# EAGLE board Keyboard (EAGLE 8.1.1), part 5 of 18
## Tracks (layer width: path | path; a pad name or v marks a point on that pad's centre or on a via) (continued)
S$4259 (continued)
  Bottom 0: 29.64,10.47 29.58,10.45
S$4260
  Bottom 0: 29.58,10.45 29.52,10.41
S$4261
  Bottom 0: 29.52,10.41 29.47,10.37
S$4262
  Bottom 0: 29.47,10.37 22.33,3.23
S$4263
  Bottom 0: 22.33,3.23 18.7,3.23
S$4264
  Bottom 0: 21.59,6.04 22.1,6.04
S$4265
  Bottom 0: 22.1,6.04 22.61,6.12
S$4266
  Bottom 0: 22.61,6.12 23.11,6.29
S$4267
  Bottom 0: 23.11,6.29 23.56,6.54
S$4268
  Bottom 0: 23.56,6.54 23.97,6.86
S$4269
  Bottom 0: 23.97,6.86 24.32,7.24
S$4270
  Bottom 0: 24.32,7.24 24.61,7.67
S$4271
  Bottom 0: 24.61,7.67 24.81,8.15
S$4272
  Bottom 0: 24.81,8.15 24.94,8.64
S$4273
  Bottom 0: 24.94,8.64 24.98,9.16
S$4274
  Bottom 0: 24.98,9.16 24.94,9.68
S$4275
  Bottom 0: 24.94,9.68 24.81,10.18
S$4276
  Bottom 0: 24.81,10.18 24.61,10.65
S$4277
  Bottom 0: 24.61,10.65 24.32,11.09
S$4278
  Bottom 0: 24.32,11.09 23.97,11.47
S$4279
  Bottom 0: 23.97,11.47 23.56,11.79
S$4280
  Bottom 0: 23.56,11.79 23.11,12.03
S$4281
  Bottom 0: 23.11,12.03 22.61,12.2
S$4282
  Bottom 0: 22.61,12.2 22.1,12.29
S$4283
  Bottom 0: 22.1,12.29 21.59,12.29
S$4284
  Bottom 0: 21.59,12.29 21.08,12.2
S$4285
  Bottom 0: 21.08,12.2 20.59,12.03
S$4286
  Bottom 0: 20.59,12.03 20.13,11.79
S$4287
  Bottom 0: 20.13,11.79 19.72,11.47
S$4288
  Bottom 0: 19.72,11.47 19.37,11.09
S$4289
  Bottom 0: 19.37,11.09 19.09,10.65
S$4290
  Bottom 0: 19.09,10.65 18.88,10.18
S$4291
  Bottom 0: 18.88,10.18 18.75,9.68
S$4292
  Bottom 0: 18.75,9.68 18.71,9.16
S$4293
  Bottom 0: 18.71,9.16 18.75,8.64
S$4294
  Bottom 0: 18.75,8.64 18.88,8.15
S$4295
  Bottom 0: 18.88,8.15 19.09,7.67
S$4296
  Bottom 0: 19.09,7.67 19.37,7.24
S$4297
  Bottom 0: 19.37,7.24 19.72,6.86
S$4298
  Bottom 0: 19.72,6.86 20.13,6.54
S$4299
  Bottom 0: 20.13,6.54 20.59,6.29
S$4300
  Bottom 0: 20.59,6.29 21.08,6.12
S$4301
  Bottom 0: 21.08,6.12 21.59,6.04
S$4302
  Bottom 0: 31.59,11.49 33.37,11.49
S$4303
  Bottom 0: 33.37,11.49 33.44,11.5
S$4304
  Bottom 0: 33.44,11.5 33.51,11.54
S$4305
  Bottom 0: 33.51,11.54 33.57,11.6
S$4306
  Bottom 0: 33.57,11.6 33.61,11.67
S$4307
  Bottom 0: 33.61,11.67 33.62,11.75
S$4308
  Bottom 0: 33.62,11.75 33.62,13.53
S$4309
  Bottom 0: 33.62,13.53 33.61,13.6
S$4310
  Bottom 0: 33.61,13.6 33.57,13.67
S$4311
  Bottom 0: 33.57,13.67 33.51,13.73
S$4312
  Bottom 0: 33.51,13.73 33.44,13.77
S$4313
  Bottom 0: 33.44,13.77 33.37,13.78
S$4314
  Bottom 0: 33.37,13.78 31.59,13.78
S$4315
  Bottom 0: 31.59,13.78 31.51,13.77
S$4316
  Bottom 0: 31.51,13.77 31.44,13.73
S$4317
  Bottom 0: 31.44,13.73 31.39,13.67
S$4318
  Bottom 0: 31.39,13.67 31.35,13.6
S$4319
  Bottom 0: 31.35,13.6 31.34,13.53
S$4320
  Bottom 0: 31.34,13.53 31.34,11.75
S$4321
  Bottom 0: 31.34,11.75 31.35,11.67
S$4322
  Bottom 0: 31.35,11.67 31.39,11.6
S$4323
  Bottom 0: 31.39,11.6 31.44,11.54
S$4324
  Bottom 0: 31.44,11.54 31.51,11.5
S$4325
  Bottom 0: 31.51,11.5 31.59,11.49
S$4326
  Bottom 0: 206.63,3.26 205.49,4.4
S$4327
  Bottom 0: 205.49,4.4 205.6,4.67
S$4328
  Bottom 0: 205.6,4.67 205.65,5.02
S$4329
  Bottom 0: 205.65,5.02 205.6,5.36
S$4330
  Bottom 0: 205.6,5.36 205.47,5.69
S$4331
  Bottom 0: 205.47,5.69 205.26,5.97
S$4332
  Bottom 0: 205.26,5.97 205,6.2
S$4333
  Bottom 0: 205,6.2 204.69,6.34
S$4334
  Bottom 0: 204.69,6.34 204.69,11.95
S$4335
  Bottom 0: 204.69,11.95 204.68,12.02
S$4336
  Bottom 0: 204.68,12.02 204.67,12.09
S$4337
  Bottom 0: 204.67,12.09 204.65,12.15
S$4338
  Bottom 0: 204.65,12.15 204.6,12.21
S$4339
  Bottom 0: 204.6,12.21 204.56,12.27
S$4340
  Bottom 0: 204.56,12.27 197.05,19.77
S$4341
  Bottom 0: 197.05,19.77 197,19.81
S$4342
  Bottom 0: 197,19.81 196.94,19.85
S$4343
  Bottom 0: 196.94,19.85 196.88,19.88
S$4344
  Bottom 0: 196.88,19.88 196.81,19.89
S$4345
  Bottom 0: 196.81,19.89 196.74,19.9
S$4346
  Bottom 0: 196.74,19.9 192.38,19.9
S$4347
  Bottom 0: 192.38,19.9 188.82,23.45
S$4348
  Bottom 0: 188.82,23.45 188.93,23.72
S$4349
  Bottom 0: 188.93,23.72 188.97,24.07
S$4350
  Bottom 0: 188.97,24.07 188.93,24.41
S$4351
  Bottom 0: 188.93,24.41 188.8,24.74
S$4352
  Bottom 0: 188.8,24.74 188.59,25.02
S$4353
  Bottom 0: 188.59,25.02 188.32,25.25
S$4354
  Bottom 0: 188.32,25.25 188.01,25.4
S$4355
  Bottom 0: 188.01,25.4 187.66,25.46
S$4356
  Bottom 0: 187.66,25.46 187.31,25.44
S$4357
  Bottom 0: 187.31,25.44
S$4358
  Bottom 0: 187.31,25.44 192.08,30.21
S$4359
  Bottom 0: 192.08,30.21 192.39,30.21
S$4360
  Bottom 0: 192.39,30.21 192.56,29.96
S$4361
  Bottom 0: 192.56,29.96 192.8,29.77
S$4362
  Bottom 0: 192.8,29.77 193.08,29.66
S$4363
  Bottom 0: 193.08,29.66 193.38,29.64
S$4364
  Bottom 0: 193.38,29.64 193.68,29.7
S$4365
  Bottom 0: 193.68,29.7 193.94,29.86
S$4366
  Bottom 0: 193.94,29.86 194.14,30.08
S$4367
  Bottom 0: 194.14,30.08 194.27,30.35
S$4368
  Bottom 0: 194.27,30.35 194.32,30.65
S$4369
  Bottom 0: 194.32,30.65 194.27,30.95
S$4370
  Bottom 0: 194.27,30.95 194.14,31.22
S$4371
  Bottom 0: 194.14,31.22 193.94,31.44
S$4372
  Bottom 0: 193.94,31.44 193.68,31.59
S$4373
  Bottom 0: 193.68,31.59 193.38,31.66
S$4374
  Bottom 0: 193.38,31.66 193.21,31.65
S$4375
  Bottom 0: 193.21,31.65 197.37,35.82
S$4376
  Bottom 0: 197.37,35.82 198.23,35.82
S$4377
  Bottom 0: 198.23,35.82 198.1,35.69
S$4378
  Bottom 0: 198.1,35.69 197.93,35.41
S$4379
  Bottom 0: 197.93,35.41 197.84,35.1
S$4380
  Bottom 0: 197.84,35.1 197.84,34.77
S$4381
  Bottom 0: 197.84,34.77 197.93,34.46
S$4382
  Bottom 0: 197.93,34.46 198.1,34.19
S$4383
  Bottom 0: 198.1,34.19 198.33,33.96
S$4384
  Bottom 0: 198.33,33.96 198.62,33.81
S$4385
  Bottom 0: 198.62,33.81 198.95,33.75
S$4386
  Bottom 0: 198.95,33.75 199.27,33.77
S$4387
  Bottom 0: 199.27,33.77 199.49,33.85
S$4388
  Bottom 0: 199.49,33.85 200.55,32.8
S$4389
  Bottom 0: 200.55,32.8 200.51,32.78
S$4390
  Bottom 0: 200.51,32.78 200.45,32.72
S$4391
  Bottom 0: 200.45,32.72 200.41,32.65
S$4392
  Bottom 0: 200.41,32.65 200.4,32.58
S$4393
  Bottom 0: 200.4,32.58 200.4,30.8
S$4394
  Bottom 0: 200.4,30.8 200.41,30.72
S$4395
  Bottom 0: 200.41,30.72 200.45,30.65
S$4396
  Bottom 0: 200.45,30.65 200.51,30.59
S$4397
  Bottom 0: 200.51,30.59 200.58,30.55
S$4398
  Bottom 0: 200.58,30.55 200.66,30.54
S$4399
  Bottom 0: 200.66,30.54 202.44,30.54
S$4400
  Bottom 0: 202.44,30.54 202.51,30.55
S$4401
  Bottom 0: 202.51,30.55 202.58,30.59
S$4402
  Bottom 0: 202.58,30.59 202.64,30.65
S$4403
  Bottom 0: 202.64,30.65 202.68,30.72
S$4404
  Bottom 0: 202.68,30.72 202.69,30.8
S$4405
  Bottom 0: 202.69,30.8 202.69,32.58
S$4406
  Bottom 0: 202.69,32.58 202.68,32.64
S$4407
  Bottom 0: 202.68,32.64 203.09,32.23
S$4408
  Bottom 0: 203.09,32.23 202.99,32.01
S$4409
  Bottom 0: 202.99,32.01 202.94,31.69
S$4410
  Bottom 0: 202.94,31.69 202.99,31.37
S$4411
  Bottom 0: 202.99,31.37 203.13,31.07
S$4412
  Bottom 0: 203.13,31.07 203.34,30.82
S$4413
  Bottom 0: 203.34,30.82 203.61,30.64
S$4414
  Bottom 0: 203.61,30.64 203.92,30.55
S$4415
  Bottom 0: 203.92,30.55 204.25,30.55
S$4416
  Bottom 0: 204.25,30.55 204.56,30.64
S$4417
  Bottom 0: 204.56,30.64 204.83,30.82
S$4418
  Bottom 0: 204.83,30.82 205.05,31.07
S$4419
  Bottom 0: 205.05,31.07 205.18,31.37
S$4420
  Bottom 0: 205.18,31.37 205.23,31.69
S$4421
  Bottom 0: 205.23,31.69 205.18,32.01
S$4422
  Bottom 0: 205.18,32.01 205.05,32.31
S$4423
  Bottom 0: 205.05,32.31 204.83,32.55
S$4424
  Bottom 0: 204.83,32.55 204.56,32.73
S$4425
  Bottom 0: 204.56,32.73 204.25,32.82
S$4426
  Bottom 0: 204.25,32.82 204.1,32.82
S$4427
  Bottom 0: 204.1,32.82 200.13,36.79
S$4428
  Bottom 0: 200.13,36.79 200.07,36.85
S$4429
  Bottom 0: 200.07,36.85 199.99,36.89
S$4430
  Bottom 0: 199.99,36.89 199.91,36.93
S$4431
  Bottom 0: 199.91,36.93 199.82,36.95
S$4432
  Bottom 0: 199.82,36.95 199.73,36.95
S$4433
  Bottom 0: 199.73,36.95 199.51,36.95
S$4434
  Bottom 0: 199.51,36.95 199.51,46.35
S$4435
  Bottom 0: 199.51,46.35 199.51,46.44
S$4436
  Bottom 0: 199.51,46.44 199.49,46.53
S$4437
  Bottom 0: 199.49,46.53 199.45,46.61
S$4438
  Bottom 0: 199.45,46.61 199.41,46.69
S$4439
  Bottom 0: 199.41,46.69 199.35,46.75
S$4440
  Bottom 0: 199.35,46.75 195.66,50.43
S$4441
  Bottom 0: 195.66,50.43 195.7,50.74
S$4442
  Bottom 0: 195.7,50.74 195.66,51.06
S$4443
  Bottom 0: 195.66,51.06 195.52,51.36
S$4444
  Bottom 0: 195.52,51.36 195.31,51.6
S$4445
  Bottom 0: 195.31,51.6 195.03,51.78
S$4446
  Bottom 0: 195.03,51.78 195,51.79
S$4447
  Bottom 0: 195,51.79 195.25,51.79
S$4448
  Bottom 0: 195.25,51.79 206.08,40.96
S$4449
  Bottom 0: 206.08,40.96 206.08,35.97
S$4450
  Bottom 0: 206.08,35.97 205.95,35.91
S$4451
  Bottom 0: 205.95,35.91 205.72,35.69
S$4452
  Bottom 0: 205.72,35.69 205.55,35.41
S$4453
  Bottom 0: 205.55,35.41 205.46,35.1
S$4454
  Bottom 0: 205.46,35.1 205.46,34.77
S$4455
  Bottom 0: 205.46,34.77 205.55,34.46
S$4456
  Bottom 0: 205.55,34.46 205.72,34.19
S$4457
  Bottom 0: 205.72,34.19 205.95,33.96
S$4458
  Bottom 0: 205.95,33.96 206.08,33.9
S$4459
  Bottom 0: 206.08,33.9 206.08,27.1
S$4460
  Bottom 0: 206.08,27.1 205.02,26.04
S$4461
  Bottom 0: 205.02,26.04 205.06,26.16
S$4462
  Bottom 0: 205.06,26.16 205.1,26.61
S$4463
  Bottom 0: 205.1,26.61 205.06,27.05
S$4464
  Bottom 0: 205.06,27.05 204.93,27.48
S$4465
  Bottom 0: 204.93,27.48 204.72,27.88
S$4466
  Bottom 0: 204.72,27.88 204.43,28.22
S$4467
  Bottom 0: 204.43,28.22 204.09,28.51
S$4468
  Bottom 0: 204.09,28.51 203.69,28.72
S$4469
  Bottom 0: 203.69,28.72 203.26,28.85
S$4470
  Bottom 0: 203.26,28.85 202.82,28.89
S$4471
  Bottom 0: 202.82,28.89 202.37,28.85
S$4472
  Bottom 0: 202.37,28.85 201.94,28.72
S$4473
  Bottom 0: 201.94,28.72 201.55,28.51
S$4474
  Bottom 0: 201.55,28.51 201.2,28.22
S$4475
  Bottom 0: 201.2,28.22 200.92,27.88
S$4476
  Bottom 0: 200.92,27.88 200.7,27.48
S$4477
  Bottom 0: 200.7,27.48 200.58,27.05
S$4478
  Bottom 0: 200.58,27.05 200.53,26.61
S$4479
  Bottom 0: 200.53,26.61 200.58,26.16
S$4480
  Bottom 0: 200.58,26.16 200.7,25.73
S$4481
  Bottom 0: 200.7,25.73 200.92,25.34
S$4482
  Bottom 0: 200.92,25.34 201.2,24.99
S$4483
  Bottom 0: 201.2,24.99 201.55,24.71
S$4484
  Bottom 0: 201.55,24.71 201.94,24.49
S$4485
  Bottom 0: 201.94,24.49 202.37,24.37
S$4486
  Bottom 0: 202.37,24.37 202.82,24.32
S$4487
  Bottom 0: 202.82,24.32 203.26,24.37
S$4488
  Bottom 0: 203.26,24.37 203.69,24.49
S$4489
  Bottom 0: 203.69,24.49 203.7,24.5
S$4490
  Bottom 0: 203.7,24.5 203.7,16.92
S$4491
  Bottom 0: 203.7,16.92 203.58,16.86
S$4492
  Bottom 0: 203.58,16.86 203.34,16.64
S$4493
  Bottom 0: 203.34,16.64 203.17,16.36
S$4494
  Bottom 0: 203.17,16.36 203.09,16.05
S$4495
  Bottom 0: 203.09,16.05 203.09,15.72
S$4496
  Bottom 0: 203.09,15.72 203.17,15.41
S$4497
  Bottom 0: 203.17,15.41 203.34,15.14
S$4498
  Bottom 0: 203.34,15.14 203.58,14.91
S$4499
  Bottom 0: 203.58,14.91 203.87,14.77
S$4500
  Bottom 0: 203.87,14.77 204.19,14.7
S$4501
  Bottom 0: 204.19,14.7 204.51,14.72
S$4502
  Bottom 0: 204.51,14.72 204.81,14.83
S$4503
  Bottom 0: 204.81,14.83 205.08,15.01
S$4504
  Bottom 0: 205.08,15.01 205.29,15.27
S$4505
  Bottom 0: 205.29,15.27 205.42,15.57
S$4506
  Bottom 0: 205.42,15.57 205.46,15.89
S$4507
  Bottom 0: 205.46,15.89 205.42,16.21
S$4508
  Bottom 0: 205.42,16.21 205.29,16.51
S$4509
  Bottom 0: 205.29,16.51 205.08,16.76
S$4510
  Bottom 0: 205.08,16.76 204.84,16.93
S$4511
  Bottom 0: 204.84,16.93 204.84,24.25
S$4512
  Bottom 0: 204.84,24.25 207.05,26.46
S$4513
  Bottom 0: 207.05,26.46 207.11,26.53
S$4514
  Bottom 0: 207.11,26.53 207.16,26.61
S$4515
  Bottom 0: 207.16,26.61 207.19,26.69
S$4516
  Bottom 0: 207.19,26.69 207.21,26.78
S$4517
  Bottom 0: 207.21,26.78 207.22,26.87
S$4518
  Bottom 0: 207.22,26.87 207.22,33.89
S$4519
  Bottom 0: 207.22,33.89 207.46,34.06
S$4520
  Bottom 0: 207.46,34.06 207.57,34.2
S$4521
  Bottom 0: 207.57,34.2 207.57,25.64
S$4522
  Bottom 0: 207.57,25.64 207.24,25.31
S$4523
  Bottom 0: 207.24,25.31 207.06,25.4
S$4524
  Bottom 0: 207.06,25.4 206.71,25.46
S$4525
  Bottom 0: 206.71,25.46 206.36,25.44
S$4526
  Bottom 0: 206.36,25.44 206.03,25.33
S$4527
  Bottom 0: 206.03,25.33 205.74,25.14
S$4528
  Bottom 0: 205.74,25.14 205.5,24.89
S$4529
  Bottom 0: 205.5,24.89 205.32,24.58
S$4530
  Bottom 0: 205.32,24.58 205.24,24.24
S$4531
  Bottom 0: 205.24,24.24 205.24,23.89
S$4532
  Bottom 0: 205.24,23.89 205.32,23.55
S$4533
  Bottom 0: 205.32,23.55 205.5,23.24
S$4534
  Bottom 0: 205.5,23.24 205.74,22.99
S$4535
  Bottom 0: 205.74,22.99 206.03,22.8
S$4536
  Bottom 0: 206.03,22.8 206.36,22.7
S$4537
  Bottom 0: 206.36,22.7 206.71,22.68
S$4538
  Bottom 0: 206.71,22.68 207.06,22.74
S$4539
  Bottom 0: 207.06,22.74 207.24,22.82
S$4540
  Bottom 0: 207.24,22.82 219.15,10.92
S$4541
  Bottom 0: 219.15,10.92 219.21,10.88
S$4542
  Bottom 0: 219.21,10.88 219.27,10.84
S$4543
  Bottom 0: 219.27,10.84 219.33,10.81
S$4544
  Bottom 0: 219.33,10.81 219.39,10.8
S$4545
  Bottom 0: 219.39,10.8 219.46,10.79
S$4546
  Bottom 0: 219.46,10.79 224.05,10.79
S$4547
  Bottom 0: 224.05,10.79 225.25,9.6
S$4548
  Bottom 0: 225.25,9.6 225.12,9.67
S$4549
  Bottom 0: 225.12,9.67 224.7,9.8
S$4550
  Bottom 0: 224.7,9.8 224.25,9.84
S$4551
  Bottom 0: 224.25,9.84 223.8,9.8
S$4552
  Bottom 0: 223.8,9.8 223.38,9.67
S$4553
  Bottom 0: 223.38,9.67 222.98,9.46
S$4554
  Bottom 0: 222.98,9.46 222.63,9.17
S$4555
  Bottom 0: 222.63,9.17 222.35,8.83
S$4556
  Bottom 0: 222.35,8.83 222.14,8.43
S$4557
  Bottom 0: 222.14,8.43 222.01,8
S$4558
  Bottom 0: 222.01,8 221.96,7.56
S$4559
  Bottom 0: 221.96,7.56 222.01,7.11
S$4560
  Bottom 0: 222.01,7.11 222.14,6.68
S$4561
  Bottom 0: 222.14,6.68 222.35,6.29
S$4562
  Bottom 0: 222.35,6.29 222.63,5.94
S$4563
  Bottom 0: 222.63,5.94 222.98,5.66
S$4564
  Bottom 0: 222.98,5.66 223.38,5.44
S$4565
  Bottom 0: 223.38,5.44 223.8,5.32
S$4566
  Bottom 0: 223.8,5.32 224.25,5.27
S$4567
  Bottom 0: 224.25,5.27 224.7,5.32
S$4568
  Bottom 0: 224.7,5.32 225.12,5.44
S$4569
  Bottom 0: 225.12,5.44 225.52,5.66
S$4570
  Bottom 0: 225.52,5.66 225.86,5.94
S$4571
  Bottom 0: 225.86,5.94 226.15,6.29
S$4572
  Bottom 0: 226.15,6.29 226.36,6.68
S$4573
  Bottom 0: 226.36,6.68 226.49,7.11
S$4574
  Bottom 0: 226.49,7.11 226.53,7.56
S$4575
  Bottom 0: 226.53,7.56 226.49,8
S$4576
  Bottom 0: 226.49,8 226.36,8.43
S$4577
  Bottom 0: 226.36,8.43 226.3,8.55
S$4578
  Bottom 0: 226.3,8.55 227.62,7.23
S$4579
  Bottom 0: 227.62,7.23 227.62,6.33
S$4580
  Bottom 0: 227.62,6.33 227.47,6.28
S$4581
  Bottom 0: 227.47,6.28 227.17,6.09
S$4582
  Bottom 0: 227.17,6.09 226.93,5.84
S$4583
  Bottom 0: 226.93,5.84 226.76,5.53
S$4584
  Bottom 0: 226.76,5.53 226.67,5.19
S$4585
  Bottom 0: 226.67,5.19 226.67,4.84
S$4586
  Bottom 0: 226.67,4.84 226.76,4.5
S$4587
  Bottom 0: 226.76,4.5 226.93,4.19
S$4588
  Bottom 0: 226.93,4.19 227.17,3.94
S$4589
  Bottom 0: 227.17,3.94 227.27,3.88
S$4590
  Bottom 0: 227.27,3.88 225.16,3.88
S$4591
  Bottom 0: 225.16,3.88 224.66,4.39
S$4592
  Bottom 0: 224.66,4.39 224.6,4.43
S$4593
  Bottom 0: 224.6,4.43 224.54,4.47
S$4594
  Bottom 0: 224.54,4.47 224.48,4.49
S$4595
  Bottom 0: 224.48,4.49 224.41,4.51
S$4596
  Bottom 0: 224.41,4.51 224.34,4.51
S$4597
  Bottom 0: 224.34,4.51 217.05,4.51
S$4598
  Bottom 0: 217.05,4.51 216.97,4.51
S$4599
  Bottom 0: 216.97,4.51 216.91,4.49
S$4600
  Bottom 0: 216.91,4.49 216.84,4.46
S$4601
  Bottom 0: 216.84,4.46 216.79,4.43
S$4602
  Bottom 0: 216.79,4.43 216.73,4.38
S$4603
  Bottom 0: 216.73,4.38 215.62,3.26
S$4604
  Bottom 0: 215.62,3.26 215.46,3.26
S$4605
  Bottom 0: 215.46,3.26 215.58,3.4
S$4606
  Bottom 0: 215.58,3.4 215.72,3.67
S$4607
  Bottom 0: 215.72,3.67 215.76,3.98
S$4608
  Bottom 0: 215.76,3.98 215.72,4.28
S$4609
  Bottom 0: 215.72,4.28 215.58,4.55
S$4610
  Bottom 0: 215.58,4.55 215.38,4.77
S$4611
  Bottom 0: 215.38,4.77 215.12,4.92
S$4612
  Bottom 0: 215.12,4.92 214.82,4.99
S$4613
  Bottom 0: 214.82,4.99 214.52,4.97
S$4614
  Bottom 0: 214.52,4.97 214.24,4.85
S$4615
  Bottom 0: 214.24,4.85 214,4.67
S$4616
  Bottom 0: 214,4.67 213.83,4.42
S$4617
  Bottom 0: 213.83,4.42 213.74,4.13
S$4618
  Bottom 0: 213.74,4.13 213.74,3.82
S$4619
  Bottom 0: 213.74,3.82 213.83,3.53
S$4620
  Bottom 0: 213.83,3.53 214,3.28
S$4621
  Bottom 0: 214,3.28 214.02,3.26
S$4622
  Bottom 0: 214.02,3.26 206.63,3.26
S$4623
  Bottom 0: 214.82,10.58 215.12,10.65
S$4624
  Bottom 0: 215.12,10.65 215.38,10.8
S$4625
  Bottom 0: 215.38,10.8 215.58,11.02
S$4626
  Bottom 0: 215.58,11.02 215.72,11.29
S$4627
  Bottom 0: 215.72,11.29 215.76,11.6
S$4628
  Bottom 0: 215.76,11.6 215.72,11.89
S$4629
  Bottom 0: 215.72,11.89 215.58,12.17
S$4630
  Bottom 0: 215.58,12.17 215.38,12.39
S$4631
  Bottom 0: 215.38,12.39 215.12,12.54
S$4632
  Bottom 0: 215.12,12.54 214.82,12.61
S$4633
  Bottom 0: 214.82,12.61 214.52,12.59
S$4634
  Bottom 0: 214.52,12.59 214.24,12.47
S$4635
  Bottom 0: 214.24,12.47 214,12.29
S$4636
  Bottom 0: 214,12.29 213.83,12.04
S$4637
  Bottom 0: 213.83,12.04 213.74,11.75
S$4638
  Bottom 0: 213.74,11.75 213.74,11.44
S$4639
  Bottom 0: 213.74,11.44 213.83,11.15
S$4640
  Bottom 0: 213.83,11.15 214,10.9
S$4641
  Bottom 0: 214,10.9 214.24,10.72
S$4642
  Bottom 0: 214.24,10.72 214.52,10.6
S$4643
  Bottom 0: 214.52,10.6 214.82,10.58
S$4644
  Bottom 0: 200.36,20.14 200.71,20.2
S$4645
  Bottom 0: 200.71,20.2 201.02,20.35
S$4646
  Bottom 0: 201.02,20.35 201.29,20.57
S$4647
  Bottom 0: 201.29,20.57 201.5,20.86
S$4648
  Bottom 0: 201.5,20.86 201.63,21.18
S$4649
  Bottom 0: 201.63,21.18 201.67,21.53
S$4650
  Bottom 0: 201.67,21.53 201.63,21.87
S$4651
  Bottom 0: 201.63,21.87 201.5,22.2
S$4652
  Bottom 0: 201.5,22.2 201.29,22.48
S$4653
  Bottom 0: 201.29,22.48 201.02,22.7
S$4654
  Bottom 0: 201.02,22.7 200.71,22.86
S$4655
  Bottom 0: 200.71,22.86 200.36,22.92
S$4656
  Bottom 0: 200.36,22.92 200.01,22.9
S$4657
  Bottom 0: 200.01,22.9 199.68,22.79
S$4658
  Bottom 0: 199.68,22.79 199.66,22.78
S$4659
  Bottom 0: 199.66,22.78 199.09,23.34
S$4660
  Bottom 0: 199.09,23.34 199.03,23.39
S$4661
  Bottom 0: 199.03,23.39 198.97,23.43
S$4662
  Bottom 0: 198.97,23.43 198.91,23.45
S$4663
  Bottom 0: 198.91,23.45 198.84,23.47
S$4664
  Bottom 0: 198.84,23.47 198.77,23.47
S$4665
  Bottom 0: 198.77,23.47 194.21,23.47
S$4666
  Bottom 0: 194.21,23.47 194.14,23.6
S$4667
  Bottom 0: 194.14,23.6 193.94,23.82
S$4668
  Bottom 0: 193.94,23.82 193.68,23.98
S$4669
  Bottom 0: 193.68,23.98 193.38,24.04
S$4670
  Bottom 0: 193.38,24.04 193.08,24.02
S$4671
  Bottom 0: 193.08,24.02 192.8,23.91
S$4672
  Bottom 0: 192.8,23.91 192.56,23.72
S$4673
  Bottom 0: 192.56,23.72 192.39,23.47
S$4674
  Bottom 0: 192.39,23.47 192.3,23.18
S$4675
  Bottom 0: 192.3,23.18 192.3,22.88
S$4676
  Bottom 0: 192.3,22.88 192.39,22.59
S$4677
  Bottom 0: 192.39,22.59 192.56,22.34
S$4678
  Bottom 0: 192.56,22.34 192.8,22.15
S$4679
  Bottom 0: 192.8,22.15 193.08,22.04
S$4680
  Bottom 0: 193.08,22.04 193.38,22.02
S$4681
  Bottom 0: 193.38,22.02 193.68,22.09
S$4682
  Bottom 0: 193.68,22.09 193.94,22.24
S$4683
  Bottom 0: 193.94,22.24 194.14,22.46
S$4684
  Bottom 0: 194.14,22.46 194.21,22.59
S$4685
  Bottom 0: 194.21,22.59 198.59,22.59
S$4686
  Bottom 0: 198.59,22.59 199.03,22.14
S$4687
  Bottom 0: 199.03,22.14 198.97,22.04
S$4688
  Bottom 0: 198.97,22.04 198.89,21.7
S$4689
  Bottom 0: 198.89,21.7 198.89,21.35
S$4690
  Bottom 0: 198.89,21.35 198.97,21.01
S$4691
  Bottom 0: 198.97,21.01 199.15,20.7
S$4692
  Bottom 0: 199.15,20.7 199.39,20.45
S$4693
  Bottom 0: 199.39,20.45 199.68,20.26
S$4694
  Bottom 0: 199.68,20.26 200.01,20.16
S$4695
  Bottom 0: 200.01,20.16 200.36,20.14
S$4696
  Bottom 0: 202.91,41.07 203.21,41.13
S$4697
  Bottom 0: 203.21,41.13 203.47,41.28
S$4698
  Bottom 0: 203.47,41.28 203.67,41.51
S$4699
  Bottom 0: 203.67,41.51 203.81,41.78
S$4700
  Bottom 0: 203.81,41.78 203.85,42.08
S$4701
  Bottom 0: 203.85,42.08 203.81,42.38
S$4702
  Bottom 0: 203.81,42.38 203.67,42.65
S$4703
  Bottom 0: 203.67,42.65 203.47,42.87
S$4704
  Bottom 0: 203.47,42.87 203.21,43.02
S$4705
  Bottom 0: 203.21,43.02 202.91,43.09
S$4706
  Bottom 0: 202.91,43.09 202.61,43.07
S$4707
  Bottom 0: 202.61,43.07 202.33,42.96
S$4708
  Bottom 0: 202.33,42.96 202.09,42.77
S$4709
  Bottom 0: 202.09,42.77 201.92,42.52
S$4710
  Bottom 0: 201.92,42.52 201.83,42.23
S$4711
  Bottom 0: 201.83,42.23 201.83,41.92
S$4712
  Bottom 0: 201.83,41.92 201.92,41.64
S$4713
  Bottom 0: 201.92,41.64 202.09,41.39
S$4714
  Bottom 0: 202.09,41.39 202.33,41.2
S$4715
  Bottom 0: 202.33,41.2 202.61,41.09
S$4716
  Bottom 0: 202.61,41.09 202.91,41.07
S$4717
  Bottom 0: 57.3,3.6 54.91,5.99
S$4718
  Bottom 0: 54.91,5.99 54.86,6.03
S$4719
  Bottom 0: 54.86,6.03 54.8,6.07
S$4720
  Bottom 0: 54.8,6.07 54.73,6.09
S$4721
  Bottom 0: 54.73,6.09 54.67,6.11
S$4722
  Bottom 0: 54.67,6.11 54.6,6.11
S$4723
  Bottom 0: 54.6,6.11 38.4,6.11
S$4724
  Bottom 0: 38.4,6.11 38.3,6.2
S$4725
  Bottom 0: 38.3,6.2 37.99,6.35
S$4726
  Bottom 0: 37.99,6.35 37.65,6.41
S$4727
  Bottom 0: 37.65,6.41 37.3,6.39
S$4728
  Bottom 0: 37.3,6.39 36.96,6.28
S$4729
  Bottom 0: 36.96,6.28 36.67,6.09
S$4730
  Bottom 0: 36.67,6.09 36.43,5.84
S$4731
  Bottom 0: 36.43,5.84 36.26,5.53
S$4732
  Bottom 0: 36.26,5.53 36.24,5.46
S$4733
  Bottom 0: 36.24,5.46 34.65,5.46
S$4734
  Bottom 0: 34.65,5.46 35.02,5.66
S$4735
  Bottom 0: 35.02,5.66 35.36,5.94
S$4736
  Bottom 0: 35.36,5.94 35.65,6.29
S$4737
  Bottom 0: 35.65,6.29 35.86,6.68
S$4738
  Bottom 0: 35.86,6.68 35.99,7.11
S$4739
  Bottom 0: 35.99,7.11 36.03,7.56
S$4740
  Bottom 0: 36.03,7.56 35.99,8
S$4741
  Bottom 0: 35.99,8 35.86,8.43
S$4742
  Bottom 0: 35.86,8.43 35.65,8.83
S$4743
  Bottom 0: 35.65,8.83 35.36,9.17
S$4744
  Bottom 0: 35.36,9.17 35.02,9.46
S$4745
  Bottom 0: 35.02,9.46 34.62,9.67
S$4746
  Bottom 0: 34.62,9.67
S$4747
  Bottom 0: 34.62,9.67 34.65,9.7
S$4748
  Bottom 0: 34.65,9.7 34.71,9.74
S$4749
  Bottom 0: 34.71,9.74 37.2,12.23
S$4750
  Bottom 0: 37.2,12.23 41.28,12.23
S$4751
  Bottom 0: 41.28,12.23 41.17,12.11
S$4752
  Bottom 0: 41.17,12.11 40.99,11.84
S$4753
  Bottom 0: 40.99,11.84 40.9,11.52
S$4754
  Bottom 0: 40.9,11.52 40.9,11.2
S$4755
  Bottom 0: 40.9,11.2 40.99,10.88
S$4756
  Bottom 0: 40.99,10.88 41.17,10.61
S$4757
  Bottom 0: 41.17,10.61 41.4,10.39
S$4758
  Bottom 0: 41.4,10.39 41.69,10.24
S$4759
  Bottom 0: 41.69,10.24 42.01,10.17
S$4760
  Bottom 0: 42.01,10.17 42.33,10.19
S$4761
  Bottom 0: 42.33,10.19 42.42,10.22
S$4762
  Bottom 0: 42.42,10.22 42.75,9.9
S$4763
  Bottom 0: 42.75,9.9 42.82,9.84
S$4764
  Bottom 0: 42.82,9.84 42.89,9.79
S$4765
  Bottom 0: 42.89,9.79 42.97,9.76
S$4766
  Bottom 0: 42.97,9.76 43.06,9.74
S$4767
  Bottom 0: 43.06,9.74 43.15,9.73
S$4768
  Bottom 0: 43.15,9.73 56.89,9.73
S$4769
  Bottom 0: 56.89,9.73 56.69,9.67
S$4770
  Bottom 0: 56.69,9.67 56.29,9.46
S$4771
  Bottom 0: 56.29,9.46 55.95,9.17
S$4772
  Bottom 0: 55.95,9.17 55.66,8.83
S$4773
  Bottom 0: 55.66,8.83 55.45,8.43
S$4774
  Bottom 0: 55.45,8.43 55.32,8
S$4775
  Bottom 0: 55.32,8 55.28,7.56
S$4776
  Bottom 0: 55.28,7.56 55.32,7.11
S$4777
  Bottom 0: 55.32,7.11 55.45,6.68
S$4778
  Bottom 0: 55.45,6.68 55.66,6.29
S$4779
  Bottom 0: 55.66,6.29 55.95,5.94
S$4780
  Bottom 0: 55.95,5.94 56.29,5.66
S$4781
  Bottom 0: 56.29,5.66 56.69,5.44
S$4782
  Bottom 0: 56.69,5.44 57.12,5.32
S$4783
  Bottom 0: 57.12,5.32 57.56,5.27
S$4784
  Bottom 0: 57.56,5.27 58.01,5.32
S$4785
  Bottom 0: 58.01,5.32 58.44,5.44
S$4786
  Bottom 0: 58.44,5.44 58.83,5.66
S$4787
  Bottom 0: 58.83,5.66 59.18,5.94
S$4788
  Bottom 0: 59.18,5.94 59.46,6.29
S$4789
  Bottom 0: 59.46,6.29 59.68,6.68
S$4790
  Bottom 0: 59.68,6.68 59.8,7.11
S$4791
  Bottom 0: 59.8,7.11 59.85,7.56
S$4792
  Bottom 0: 59.85,7.56 59.8,8
S$4793
  Bottom 0: 59.8,8 59.68,8.43
S$4794
  Bottom 0: 59.68,8.43 59.46,8.83
S$4795
  Bottom 0: 59.46,8.83 59.18,9.17
S$4796
  Bottom 0: 59.18,9.17 58.83,9.46
S$4797
  Bottom 0: 58.83,9.46 58.44,9.67
S$4798
  Bottom 0: 58.44,9.67 58.23,9.73
S$4799
  Bottom 0: 58.23,9.73 58.55,9.73
S$4800
  Bottom 0: 58.55,9.73 58.65,9.74
S$4801
  Bottom 0: 58.65,9.74 58.73,9.76
S$4802
  Bottom 0: 58.73,9.76 58.81,9.79
S$4803
  Bottom 0: 58.81,9.79 58.89,9.84
S$4804
  Bottom 0: 58.89,9.84 58.96,9.9
S$4805
  Bottom 0: 58.96,9.9 61.78,12.72
S$4806
  Bottom 0: 61.78,12.72 61.84,12.78
S$4807
  Bottom 0: 61.84,12.78 61.88,12.86
S$4808
  Bottom 0: 61.88,12.86 61.92,12.94
S$4809
  Bottom 0: 61.92,12.94 61.94,13.03
S$4810
  Bottom 0: 61.94,13.03 61.95,13.12
S$4811
  Bottom 0: 61.95,13.12 61.95,14.84
S$4812
  Bottom 0: 61.95,14.84 62.19,15.01
S$4813
  Bottom 0: 62.19,15.01 62.4,15.27
S$4814
  Bottom 0: 62.4,15.27 62.52,15.57
S$4815
  Bottom 0: 62.52,15.57 62.57,15.89
S$4816
  Bottom 0: 62.57,15.89 62.52,16.21
S$4817
  Bottom 0: 62.52,16.21 62.4,16.51
S$4818
  Bottom 0: 62.4,16.51 62.19,16.76
S$4819
  Bottom 0: 62.19,16.76 61.92,16.95
S$4820
  Bottom 0: 61.92,16.95 61.62,17.06
S$4821
  Bottom 0: 61.62,17.06 61.3,17.08
S$4822
  Bottom 0: 61.3,17.08 61.04,17.03
S$4823
  Bottom 0: 61.04,17.03 59.06,19.01
S$4824
  Bottom 0: 59.06,19.01 59.06,22.54
S$4825
  Bottom 0: 59.06,22.54 59.19,22.34
S$4826
  Bottom 0: 59.19,22.34 59.43,22.15
S$4827
  Bottom 0: 59.43,22.15 59.71,22.04
S$4828
  Bottom 0: 59.71,22.04 60.02,22.02
S$4829
  Bottom 0: 60.02,22.02 60.31,22.09
S$4830
  Bottom 0: 60.31,22.09 60.58,22.24
S$4831
  Bottom 0: 60.58,22.24 60.78,22.46
S$4832
  Bottom 0: 60.78,22.46 60.84,22.59
S$4833
  Bottom 0: 60.84,22.59 65.23,22.59
S$4834
  Bottom 0: 65.23,22.59 65.68,22.14
S$4835
  Bottom 0: 65.68,22.14 65.63,22.04
S$4836
  Bottom 0: 65.63,22.04 65.54,21.7
S$4837
  Bottom 0: 65.54,21.7 65.54,21.35
S$4838
  Bottom 0: 65.54,21.35 65.63,21.01
S$4839
  Bottom 0: 65.63,21.01 65.8,20.7
S$4840
  Bottom 0: 65.8,20.7 66.04,20.45
S$4841
  Bottom 0: 66.04,20.45 66.33,20.26
S$4842
  Bottom 0: 66.33,20.26 66.66,20.16
S$4843
  Bottom 0: 66.66,20.16 67.01,20.14
S$4844
  Bottom 0: 67.01,20.14 67.36,20.2
S$4845
  Bottom 0: 67.36,20.2 67.67,20.35
S$4846
  Bottom 0: 67.67,20.35 67.94,20.57
S$4847
  Bottom 0: 67.94,20.57 68.15,20.86
S$4848
  Bottom 0: 68.15,20.86 68.28,21.18
S$4849
  Bottom 0: 68.28,21.18 68.32,21.53
S$4850
  Bottom 0: 68.32,21.53 68.28,21.87
S$4851
  Bottom 0: 68.28,21.87 68.15,22.2
S$4852
  Bottom 0: 68.15,22.2 67.94,22.48
S$4853
  Bottom 0: 67.94,22.48 67.67,22.7
S$4854
  Bottom 0: 67.67,22.7 67.36,22.86
S$4855
  Bottom 0: 67.36,22.86 67.01,22.92
S$4856
  Bottom 0: 67.01,22.92 66.66,22.9
S$4857
  Bottom 0: 66.66,22.9 66.33,22.79
S$4858
  Bottom 0: 66.33,22.79 66.3,22.78
S$4859
  Bottom 0: 66.3,22.78 65.73,23.34
S$4860
  Bottom 0: 65.73,23.34 65.68,23.39
S$4861
  Bottom 0: 65.68,23.39 65.62,23.43
S$4862
  Bottom 0: 65.62,23.43 65.56,23.45
S$4863
  Bottom 0: 65.56,23.45 65.49,23.47
S$4864
  Bottom 0: 65.49,23.47 65.42,23.47
S$4865
  Bottom 0: 65.42,23.47 60.84,23.47
S$4866
  Bottom 0: 60.84,23.47 60.78,23.6
S$4867
  Bottom 0: 60.78,23.6 60.58,23.82
S$4868
  Bottom 0: 60.58,23.82 60.31,23.98
S$4869
  Bottom 0: 60.31,23.98 60.02,24.04
S$4870
  Bottom 0: 60.02,24.04 59.71,24.02
S$4871
  Bottom 0: 59.71,24.02 59.43,23.91
S$4872
  Bottom 0: 59.43,23.91 59.19,23.72
S$4873
  Bottom 0: 59.19,23.72 59.06,23.52
S$4874
  Bottom 0: 59.06,23.52 59.06,30.16
S$4875
  Bottom 0: 59.06,30.16 59.19,29.96
S$4876
  Bottom 0: 59.19,29.96 59.43,29.77
S$4877
  Bottom 0: 59.43,29.77 59.71,29.66
S$4878
  Bottom 0: 59.71,29.66 60.02,29.64
S$4879
  Bottom 0: 60.02,29.64 60.31,29.7
S$4880
  Bottom 0: 60.31,29.7 60.58,29.86
S$4881
  Bottom 0: 60.58,29.86 60.78,30.08
S$4882
  Bottom 0: 60.78,30.08 60.91,30.35
S$4883
  Bottom 0: 60.91,30.35 60.96,30.65
S$4884
  Bottom 0: 60.96,30.65 60.91,30.95
S$4885
  Bottom 0: 60.91,30.95 60.78,31.22
S$4886
  Bottom 0: 60.78,31.22 60.58,31.44
S$4887
  Bottom 0: 60.58,31.44 60.31,31.59
S$4888
  Bottom 0: 60.31,31.59 60.02,31.66
S$4889
  Bottom 0: 60.02,31.66 59.71,31.64
S$4890
  Bottom 0: 59.71,31.64 59.43,31.53
S$4891
  Bottom 0: 59.43,31.53 59.19,31.34
S$4892
  Bottom 0: 59.19,31.34 59.03,31.09
S$4893
  Bottom 0: 59.03,31.09 58.99,30.96
S$4894
  Bottom 0: 58.99,30.96 58.95,31.02
S$4895
  Bottom 0: 58.95,31.02 58.89,31.08
S$4896
  Bottom 0: 58.89,31.08 55.38,34.6
S$4897
  Bottom 0: 55.38,34.6 55.38,34.62
S$4898
  Bottom 0: 55.38,34.62 55.42,34.94
S$4899
  Bottom 0: 55.42,34.94 55.38,35.26
S$4900
  Bottom 0: 55.38,35.26 55.25,35.56
S$4901
  Bottom 0: 55.25,35.56 55.04,35.81
S$4902
  Bottom 0: 55.04,35.81 54.78,36
S$4903
  Bottom 0: 54.78,36 54.58,36.07
S$4904
  Bottom 0: 54.58,36.07 65.31,36.07
S$4905
  Bottom 0: 65.31,36.07 65.27,36.06
S$4906
  Bottom 0: 65.27,36.06 64.97,35.91
S$4907
  Bottom 0: 64.97,35.91 64.74,35.69
S$4908
  Bottom 0: 64.74,35.69 64.57,35.41
S$4909
  Bottom 0: 64.57,35.41 64.48,35.1
S$4910
  Bottom 0: 64.48,35.1 64.48,34.77
S$4911
  Bottom 0: 64.48,34.77 64.57,34.46
S$4912
  Bottom 0: 64.57,34.46 64.74,34.19
S$4913
  Bottom 0: 64.74,34.19 64.97,33.96
S$4914
  Bottom 0: 64.97,33.96 65.27,33.81
S$4915
  Bottom 0: 65.27,33.81 65.58,33.75
S$4916
  Bottom 0: 65.58,33.75 65.91,33.77
S$4917
  Bottom 0: 65.91,33.77 66.13,33.85
S$4918
  Bottom 0: 66.13,33.85 67.18,32.79
S$4919
  Bottom 0: 67.18,32.79 67.16,32.78
S$4920
  Bottom 0: 67.16,32.78 67.1,32.72
S$4921
  Bottom 0: 67.1,32.72 67.06,32.65
S$4922
  Bottom 0: 67.06,32.65 67.05,32.58
S$4923
  Bottom 0: 67.05,32.58 67.05,30.8
S$4924
  Bottom 0: 67.05,30.8 67.06,30.72
S$4925
  Bottom 0: 67.06,30.72 67.1,30.65
S$4926
  Bottom 0: 67.1,30.65 67.16,30.59
S$4927
  Bottom 0: 67.16,30.59 67.23,30.55
S$4928
  Bottom 0: 67.23,30.55 67.31,30.54
S$4929
  Bottom 0: 67.31,30.54 69.08,30.54
S$4930
  Bottom 0: 69.08,30.54 69.14,30.55
S$4931
  Bottom 0: 69.14,30.55 71.49,28.2
S$4932
  Bottom 0: 71.49,28.2 71.49,27.65
S$4933
  Bottom 0: 71.49,27.65 71.37,27.88
S$4934
  Bottom 0: 71.37,27.88 71.08,28.22
S$4935
  Bottom 0: 71.08,28.22 70.74,28.51
S$4936
  Bottom 0: 70.74,28.51 70.34,28.72
S$4937
  Bottom 0: 70.34,28.72 69.91,28.85
S$4938
  Bottom 0: 69.91,28.85 69.47,28.89
S$4939
  Bottom 0: 69.47,28.89 69.02,28.85
S$4940
  Bottom 0: 69.02,28.85 68.59,28.72
S$4941
  Bottom 0: 68.59,28.72 68.2,28.51
S$4942
  Bottom 0: 68.2,28.51 67.85,28.22
S$4943
  Bottom 0: 67.85,28.22 67.57,27.88
S$4944
  Bottom 0: 67.57,27.88 67.35,27.48
S$4945
  Bottom 0: 67.35,27.48 67.22,27.05
S$4946
  Bottom 0: 67.22,27.05 67.18,26.61
S$4947
  Bottom 0: 67.18,26.61 67.22,26.16
S$4948
  Bottom 0: 67.22,26.16 67.35,25.73
S$4949
  Bottom 0: 67.35,25.73 67.57,25.34
S$4950
  Bottom 0: 67.57,25.34 67.85,24.99
S$4951
  Bottom 0: 67.85,24.99 68.2,24.71
S$4952
  Bottom 0: 68.2,24.71 68.59,24.49
S$4953
  Bottom 0: 68.59,24.49 69.02,24.37
S$4954
  Bottom 0: 69.02,24.37 69.47,24.32
S$4955
  Bottom 0: 69.47,24.32 69.91,24.37
S$4956
  Bottom 0: 69.91,24.37 70.23,24.46
S$4957
  Bottom 0: 70.23,24.46
S$4958
  Bottom 0: 70.23,24.46 70.19,24.4
S$4959
  Bottom 0: 70.19,24.4 70.16,24.34
S$4960
  Bottom 0: 70.16,24.34 70.14,24.27
S$4961
  Bottom 0: 70.14,24.27 70.14,24.2
S$4962
  Bottom 0: 70.14,24.2 70.14,19.28
S$4963
  Bottom 0: 70.14,19.28 70,19.12
S$4964
  Bottom 0: 70,19.12 69.91,18.89
S$4965
  Bottom 0: 69.91,18.89 69.91,18.64
S$4966
  Bottom 0: 69.91,18.64 70,18.4
S$4967
  Bottom 0: 70,18.4 70.14,18.25
S$4968
  Bottom 0: 70.14,18.25 70.14,14.42
S$4969
  Bottom 0: 70.14,14.42 61.99,6.26
S$4970
  Bottom 0: 61.99,6.26 61.81,6.35
S$4971
  Bottom 0: 61.81,6.35 61.46,6.41
S$4972
  Bottom 0: 61.46,6.41 61.11,6.39
S$4973
  Bottom 0: 61.11,6.39 60.78,6.28
S$4974
  Bottom 0: 60.78,6.28 60.48,6.09
S$4975
  Bottom 0: 60.48,6.09 60.25,5.84
S$4976
  Bottom 0: 60.25,5.84 60.07,5.53
S$4977
  Bottom 0: 60.07,5.53 59.98,5.19
S$4978
  Bottom 0: 59.98,5.19 59.98,4.84
S$4979
  Bottom 0: 59.98,4.84 60.07,4.5
S$4980
  Bottom 0: 60.07,4.5 60.25,4.19
S$4981
  Bottom 0: 60.25,4.19 60.48,3.94
S$4982
  Bottom 0: 60.48,3.94 60.78,3.75
S$4983
  Bottom 0: 60.78,3.75 61.11,3.65
S$4984
  Bottom 0: 61.11,3.65 61.46,3.62
S$4985
  Bottom 0: 61.46,3.62 61.81,3.69
S$4986
  Bottom 0: 61.81,3.69 62.12,3.84
S$4987
  Bottom 0: 62.12,3.84 62.39,4.06
S$4988
  Bottom 0: 62.39,4.06 62.6,4.35
S$4989
  Bottom 0: 62.6,4.35 62.73,4.67
S$4990
  Bottom 0: 62.73,4.67 62.77,5.02
S$4991
  Bottom 0: 62.77,5.02 62.73,5.36
S$4992
  Bottom 0: 62.73,5.36 62.62,5.63
S$4993
  Bottom 0: 62.62,5.63 70.9,13.92
S$4994
  Bottom 0: 70.9,13.92 70.94,13.97
S$4995
  Bottom 0: 70.94,13.97 70.98,14.03
S$4996
  Bottom 0: 70.98,14.03 71,14.09
S$4997
  Bottom 0: 71,14.09 71.02,14.16
S$4998
  Bottom 0: 71.02,14.16 71.03,14.23
S$4999
  Bottom 0: 71.03,14.23 71.03,18.25
S$5000
  Bottom 0: 71.03,18.25 71.09,18.3
S$5001
  Bottom 0: 71.09,18.3 71.22,18.51
S$5002
  Bottom 0: 71.22,18.51 71.27,18.76
S$5003
  Bottom 0: 71.27,18.76 71.22,19.01
S$5004
  Bottom 0: 71.22,19.01 71.09,19.23
S$5005
  Bottom 0: 71.09,19.23 71.03,19.28
S$5006
  Bottom 0: 71.03,19.28 71.03,24.01
S$5007
  Bottom 0: 71.03,24.01 72.24,25.23
S$5008
  Bottom 0: 72.24,25.23 72.29,25.29
S$5009
  Bottom 0: 72.29,25.29 72.33,25.35
S$5010
  Bottom 0: 72.33,25.35 72.35,25.41
S$5011
  Bottom 0: 72.35,25.41 72.36,25.47
S$5012
  Bottom 0: 72.36,25.47 72.37,25.55
S$5013
  Bottom 0: 72.37,25.55 72.37,28.38
S$5014
  Bottom 0: 72.37,28.38 72.36,28.46
S$5015
  Bottom 0: 72.36,28.46 72.35,28.52
S$5016
  Bottom 0: 72.35,28.52 72.33,28.58
S$5017
  Bottom 0: 72.33,28.58 72.29,28.64
S$5018
  Bottom 0: 72.29,28.64 72.24,28.7
S$5019
  Bottom 0: 72.24,28.7 70.31,30.63
S$5020
  Bottom 0: 70.31,30.63 70.57,30.55
S$5021
  Bottom 0: 70.57,30.55 70.9,30.55
S$5022
  Bottom 0: 70.9,30.55 71.03,30.59
S$5023
  Bottom 0: 71.03,30.59 75.66,25.96
S$5024
  Bottom 0: 75.66,25.96 75.66,23.28
S$5025
  Bottom 0: 75.66,23.28 75.67,23.19
S$5026
  Bottom 0: 75.67,23.19 75.69,23.1
S$5027
  Bottom 0: 75.69,23.1 75.72,23.02
S$5028
  Bottom 0: 75.72,23.02 75.77,22.94
S$5029
  Bottom 0: 75.77,22.94 75.83,22.88
S$5030
  Bottom 0: 75.83,22.88 90.94,7.76
S$5031
  Bottom 0: 90.94,7.76 90.9,7.59
S$5032
  Bottom 0: 90.9,7.59 90.9,7.27
S$5033
  Bottom 0: 90.9,7.27 90.98,6.95
S$5034
  Bottom 0: 90.98,6.95 91.16,6.68
S$5035
  Bottom 0: 91.16,6.68 91.39,6.45
S$5036
  Bottom 0: 91.39,6.45 91.68,6.31
S$5037
  Bottom 0: 91.68,6.31 92,6.24
S$5038
  Bottom 0: 92,6.24 92.33,6.26
S$5039
  Bottom 0: 92.33,6.26 92.63,6.37
S$5040
  Bottom 0: 92.63,6.37 92.89,6.56
S$5041
  Bottom 0: 92.89,6.56 93.1,6.81
S$5042
  Bottom 0: 93.1,6.81 93.23,7.11
S$5043
  Bottom 0: 93.23,7.11 93.28,7.43
S$5044
  Bottom 0: 93.28,7.43 93.23,7.75
S$5045
  Bottom 0: 93.23,7.75 93.1,8.05
S$5046
  Bottom 0: 93.1,8.05 92.89,8.3
S$5047
  Bottom 0: 92.89,8.3 92.63,8.49
S$5048
  Bottom 0: 92.63,8.49 92.33,8.6
S$5049
  Bottom 0: 92.33,8.6 92,8.62
S$5050
  Bottom 0: 92,8.62 91.75,8.57
S$5051
  Bottom 0: 91.75,8.57 76.81,23.5
S$5052
  Bottom 0: 76.81,23.5 77,23.41
S$5053
  Bottom 0: 77,23.41 77.25,23.39
S$5054
  Bottom 0: 77.25,23.39 77.5,23.45
S$5055
  Bottom 0: 77.5,23.45 77.7,23.6
S$5056
  Bottom 0: 77.7,23.6 77.83,23.82
S$5057
  Bottom 0: 77.83,23.82 77.88,24.07
S$5058
  Bottom 0: 77.88,24.07 77.83,24.32
S$5059
  Bottom 0: 77.83,24.32 77.7,24.53
S$5060
  Bottom 0: 77.7,24.53 77.63,24.58
S$5061
  Bottom 0: 77.63,24.58 77.63,32.63
S$5062
  Bottom 0: 77.63,32.63 85.74,40.74
S$5063
  Bottom 0: 85.74,40.74 85.78,40.79
S$5064
  Bottom 0: 85.78,40.79 85.82,40.85
S$5065
  Bottom 0: 85.82,40.85 85.85,40.91
S$5066
  Bottom 0: 85.85,40.91 85.86,40.98
S$5067
  Bottom 0: 85.86,40.98 85.87,41.05
S$5068
  Bottom 0: 85.87,41.05 85.87,61.73
S$5069
  Bottom 0: 85.87,61.73 95.77,61.73
S$5070
  Bottom 0: 95.77,61.73 95.79,61.65
S$5071
  Bottom 0: 95.79,61.65 95.96,61.34
S$5072
  Bottom 0: 95.96,61.34 96.2,61.09
S$5073
  Bottom 0: 96.2,61.09 96.5,60.9
S$5074
  Bottom 0: 96.5,60.9 96.83,60.8
S$5075
  Bottom 0: 96.83,60.8 97.18,60.77
S$5076
  Bottom 0: 97.18,60.77 97.52,60.84
S$5077
  Bottom 0: 97.52,60.84 97.84,60.99
S$5078
  Bottom 0: 97.84,60.99 98.11,61.21
S$5079
  Bottom 0: 98.11,61.21 98.32,61.5
S$5080
  Bottom 0: 98.32,61.5 98.44,61.82
S$5081
  Bottom 0: 98.44,61.82 98.49,62.17
S$5082
  Bottom 0: 98.49,62.17 98.44,62.51
S$5083
  Bottom 0: 98.44,62.51 98.32,62.84
S$5084
  Bottom 0: 98.32,62.84 98.11,63.12
S$5085
  Bottom 0: 98.11,63.12 97.84,63.34
S$5086
  Bottom 0: 97.84,63.34 97.52,63.5
S$5087
  Bottom 0: 97.52,63.5 97.18,63.56
S$5088
  Bottom 0: 97.18,63.56 96.83,63.54
S$5089
  Bottom 0: 96.83,63.54 96.5,63.43
S$5090
  Bottom 0: 96.5,63.43 96.2,63.24
S$5091
  Bottom 0: 96.2,63.24 95.96,62.99
S$5092
  Bottom 0: 95.96,62.99 95.79,62.68
S$5093
  Bottom 0: 95.79,62.68 95.77,62.61
S$5094
  Bottom 0: 95.77,62.61 94.18,62.61
S$5095
  Bottom 0: 94.18,62.61 94.55,62.81
S$5096
  Bottom 0: 94.55,62.81 94.9,63.09
S$5097
  Bottom 0: 94.9,63.09 95.18,63.44
S$5098
  Bottom 0: 95.18,63.44 95.39,63.83
S$5099
  Bottom 0: 95.39,63.83 95.52,64.26
S$5100
  Bottom 0: 95.52,64.26 95.57,64.71
S$5101
  Bottom 0: 95.57,64.71 95.52,65.15
S$5102
  Bottom 0: 95.52,65.15 95.39,65.58
S$5103
  Bottom 0: 95.39,65.58 95.18,65.98
S$5104
  Bottom 0: 95.18,65.98 94.9,66.32
S$5105
  Bottom 0: 94.9,66.32 94.55,66.61
S$5106
  Bottom 0: 94.55,66.61 94.16,66.82
S$5107
  Bottom 0: 94.16,66.82 93.73,66.94
S$5108
  Bottom 0: 93.73,66.94 93.28,66.99
S$5109
  Bottom 0: 93.28,66.99 92.83,66.94
S$5110
  Bottom 0: 92.83,66.94 92.41,66.82
S$5111
  Bottom 0: 92.41,66.82 92.01,66.61
S$5112
  Bottom 0: 92.01,66.61 91.67,66.32
S$5113
  Bottom 0: 91.67,66.32 91.38,65.98
S$5114
  Bottom 0: 91.38,65.98 91.17,65.58
S$5115
  Bottom 0: 91.17,65.58 91.04,65.15
S$5116
  Bottom 0: 91.04,65.15 91,64.71
S$5117
  Bottom 0: 91,64.71 91.04,64.26
S$5118
  Bottom 0: 91.04,64.26 91.17,63.83
S$5119
  Bottom 0: 91.17,63.83 91.38,63.44
S$5120
  Bottom 0: 91.38,63.44 91.67,63.09
S$5121
  Bottom 0: 91.67,63.09 92.01,62.81
S$5122
  Bottom 0: 92.01,62.81 92.38,62.61
S$5123
  Bottom 0: 92.38,62.61 85.62,62.61
S$5124
  Bottom 0: 85.62,62.61 75.12,73.11
S$5125
  Bottom 0: 75.12,73.11 75.12,74.34
S$5126
  Bottom 0: 75.12,74.34 75.19,74.39
S$5127
  Bottom 0: 75.19,74.39 75.32,74.61
S$5128
  Bottom 0: 75.32,74.61 75.36,74.86
S$5129
  Bottom 0: 75.36,74.86 75.35,74.94
S$5130
  Bottom 0: 75.35,74.94 76.91,73.38
S$5131
  Bottom 0: 76.91,73.38 76.86,73.2
S$5132
  Bottom 0: 76.86,73.2 76.86,72.88
S$5133
  Bottom 0: 76.86,72.88 76.95,72.56
S$5134
  Bottom 0: 76.95,72.56 77.12,72.29
S$5135
  Bottom 0: 77.12,72.29 77.35,72.07
S$5136
  Bottom 0: 77.35,72.07 77.64,71.92
S$5137
  Bottom 0: 77.64,71.92 77.97,71.85
S$5138
  Bottom 0: 77.97,71.85 78.29,71.87
S$5139
  Bottom 0: 78.29,71.87 78.59,71.98
S$5140
  Bottom 0: 78.59,71.98 78.86,72.17
S$5141
  Bottom 0: 78.86,72.17 79.06,72.42
S$5142
  Bottom 0: 79.06,72.42 79.09,72.47
S$5143
  Bottom 0: 79.09,72.47 85.2,72.47
S$5144
  Bottom 0: 85.2,72.47 85.29,72.48
S$5145
  Bottom 0: 85.29,72.48 85.38,72.5
S$5146
  Bottom 0: 85.38,72.5 85.46,72.53
S$5147
  Bottom 0: 85.46,72.53 85.53,72.58
S$5148
  Bottom 0: 85.53,72.58 85.6,72.64
S$5149
  Bottom 0: 85.6,72.64 87.24,74.28
S$5150
  Bottom 0: 87.24,74.28 87.5,74.23
S$5151
  Bottom 0: 87.5,74.23 87.82,74.25
S$5152
  Bottom 0: 87.82,74.25 88.12,74.36
S$5153
  Bottom 0: 88.12,74.36 88.39,74.55
S$5154
  Bottom 0: 88.39,74.55 88.59,74.8
S$5155
  Bottom 0: 88.59,74.8 88.62,74.85
S$5156
  Bottom 0: 88.62,74.85 94.49,74.85
S$5157
  Bottom 0: 94.49,74.85 95.96,73.38
S$5158
  Bottom 0: 95.96,73.38 95.92,73.2
S$5159
  Bottom 0: 95.92,73.2 95.92,72.88
S$5160
  Bottom 0: 95.92,72.88 96,72.56
S$5161
  Bottom 0: 96,72.56 96.18,72.29
S$5162
  Bottom 0: 96.18,72.29 96.41,72.07
S$5163
  Bottom 0: 96.41,72.07 96.7,71.92
S$5164
  Bottom 0: 96.7,71.92 97.02,71.85
S$5165
  Bottom 0: 97.02,71.85 97.35,71.87
S$5166
  Bottom 0: 97.35,71.87 97.65,71.98
S$5167
  Bottom 0: 97.65,71.98 97.91,72.17
S$5168
  Bottom 0: 97.91,72.17 98.12,72.42
S$5169
  Bottom 0: 98.12,72.42 98.14,72.47
S$5170
  Bottom 0: 98.14,72.47 103.52,72.47
S$5171
  Bottom 0: 103.52,72.47 103.52,69.46
S$5172
  Bottom 0: 103.52,69.46 103.45,69.54
S$5173
  Bottom 0: 103.45,69.54 103.18,69.69
S$5174
  Bottom 0: 103.18,69.69 102.89,69.76
S$5175
  Bottom 0: 102.89,69.76 102.58,69.74
S$5176
  Bottom 0: 102.58,69.74 102.3,69.63
S$5177
  Bottom 0: 102.3,69.63 102.06,69.44
S$5178
  Bottom 0: 102.06,69.44 101.89,69.19
S$5179
  Bottom 0: 101.89,69.19 101.8,68.9
S$5180
  Bottom 0: 101.8,68.9 101.8,68.75
S$5181
  Bottom 0: 101.8,68.75 95.03,68.75
S$5182
  Bottom 0: 95.03,68.75 95.3,68.92
S$5183
  Bottom 0: 95.3,68.92 95.51,69.16
S$5184
  Bottom 0: 95.51,69.16 95.65,69.47
S$5185
  Bottom 0: 95.65,69.47 95.69,69.79
S$5186
  Bottom 0: 95.69,69.79 95.65,70.11
S$5187
  Bottom 0: 95.65,70.11 95.51,70.41
S$5188
  Bottom 0: 95.51,70.41 95.3,70.65
S$5189
  Bottom 0: 95.3,70.65 95.02,70.83
S$5190
  Bottom 0: 95.02,70.83 94.71,70.92
S$5191
  Bottom 0: 94.71,70.92 94.39,70.92
S$5192
  Bottom 0: 94.39,70.92 94.08,70.83
S$5193
  Bottom 0: 94.08,70.83 93.8,70.65
S$5194
  Bottom 0: 93.8,70.65 93.59,70.41
S$5195
  Bottom 0: 93.59,70.41 93.45,70.11
S$5196
  Bottom 0: 93.45,70.11 93.41,69.79
S$5197
  Bottom 0: 93.41,69.79 93.45,69.47
S$5198
  Bottom 0: 93.45,69.47 93.59,69.16
S$5199
  Bottom 0: 93.59,69.16 93.8,68.92
S$5200
  Bottom 0: 93.8,68.92 94.07,68.75
S$5201
  Bottom 0: 94.07,68.75 93.1,68.75
S$5202
  Bottom 0: 93.1,68.75 93.14,68.82
S$5203
  Bottom 0: 93.14,68.82 93.15,68.9
S$5204
  Bottom 0: 93.15,68.9 93.15,70.67
S$5205
  Bottom 0: 93.15,70.67 93.14,70.75
S$5206
  Bottom 0: 93.14,70.75 93.1,70.82
S$5207
  Bottom 0: 93.1,70.82 93.05,70.88
S$5208
  Bottom 0: 93.05,70.88 92.97,70.92
S$5209
  Bottom 0: 92.97,70.92 92.9,70.93
S$5210
  Bottom 0: 92.9,70.93 92.45,70.93
S$5211
  Bottom 0: 92.45,70.93 92.45,71.06
S$5212
  Bottom 0: 92.45,71.06 92.39,71.28
S$5213
  Bottom 0: 92.39,71.28 92.23,71.44
S$5214
  Bottom 0: 92.23,71.44 92.01,71.5
S$5215
  Bottom 0: 92.01,71.5 91.66,71.5
S$5216
  Bottom 0: 91.66,71.5 90.57,72.59
S$5217
  Bottom 0: 90.57,72.59 90.63,72.72
S$5218
  Bottom 0: 90.63,72.72 90.67,73.04
S$5219
  Bottom 0: 90.67,73.04 90.63,73.36
S$5220
  Bottom 0: 90.63,73.36 90.5,73.66
S$5221
  Bottom 0: 90.5,73.66 90.29,73.92
S$5222
  Bottom 0: 90.29,73.92 90.03,74.11
S$5223
  Bottom 0: 90.03,74.11 89.72,74.21
S$5224
  Bottom 0: 89.72,74.21 89.4,74.23
S$5225
  Bottom 0: 89.4,74.23 89.08,74.17
S$5226
  Bottom 0: 89.08,74.17 88.79,74.02
S$5227
  Bottom 0: 88.79,74.02 88.56,73.8
S$5228
  Bottom 0: 88.56,73.8 88.38,73.52
S$5229
  Bottom 0: 88.38,73.52 88.3,73.2
S$5230
  Bottom 0: 88.3,73.2 88.3,72.88
S$5231
  Bottom 0: 88.3,72.88 88.38,72.56
S$5232
  Bottom 0: 88.38,72.56 88.56,72.29
S$5233
  Bottom 0: 88.56,72.29 88.79,72.07
S$5234
  Bottom 0: 88.79,72.07 89.08,71.92
S$5235
  Bottom 0: 89.08,71.92 89.4,71.85
S$5236
  Bottom 0: 89.4,71.85 89.72,71.87
S$5237
  Bottom 0: 89.72,71.87 89.94,71.95
S$5238
  Bottom 0: 89.94,71.95 91,70.89
S$5239
  Bottom 0: 91,70.89 90.97,70.88
S$5240
  Bottom 0: 90.97,70.88 90.92,70.82
S$5241
  Bottom 0: 90.92,70.82 90.88,70.75
S$5242
  Bottom 0: 90.88,70.75 90.87,70.67
S$5243
  Bottom 0: 90.87,70.67 90.87,68.9
S$5244
  Bottom 0: 90.87,68.9 90.88,68.82
S$5245
  Bottom 0: 90.88,68.82 90.92,68.75
S$5246
  Bottom 0: 90.92,68.75 84.78,68.75
S$5247
  Bottom 0: 84.78,68.75 84.73,69.05
S$5248
  Bottom 0: 84.73,69.05 84.6,69.32
S$5249
  Bottom 0: 84.6,69.32 84.4,69.54
S$5250
  Bottom 0: 84.4,69.54 84.13,69.69
S$5251
  Bottom 0: 84.13,69.69 83.84,69.76
S$5252
  Bottom 0: 83.84,69.76 83.53,69.74
S$5253
  Bottom 0: 83.53,69.74 83.25,69.63
S$5254
  Bottom 0: 83.25,69.63 83.02,69.44
S$5255
  Bottom 0: 83.02,69.44 82.84,69.19
S$5256
  Bottom 0: 82.84,69.19 82.75,68.9
S$5257
  Bottom 0: 82.75,68.9 82.75,68.59
S$5258
  Bottom 0: 82.75,68.59 82.84,68.31
S$5259
  Bottom 0: 82.84,68.31 83.02,68.06
S$5260
  Bottom 0: 83.02,68.06 83.25,67.87
S$5261
  Bottom 0: 83.25,67.87 83.53,67.76
S$5262
  Bottom 0: 83.53,67.76 83.84,67.74
S$5263
  Bottom 0: 83.84,67.74 84.13,67.81
S$5264
  Bottom 0: 84.13,67.81 84.24,67.87
S$5265
  Bottom 0: 84.24,67.87 102.31,67.87
S$5266
  Bottom 0: 102.31,67.87 102.58,67.76
S$5267
  Bottom 0: 102.58,67.76 102.89,67.74
S$5268
  Bottom 0: 102.89,67.74 103.18,67.81
S$5269
  Bottom 0: 103.18,67.81 103.45,67.95
S$5270
  Bottom 0: 103.45,67.95 103.52,68.04
S$5271
  Bottom 0: 103.52,68.04 103.52,61.84
S$5272
  Bottom 0: 103.52,61.84 103.45,61.92
S$5273
  Bottom 0: 103.45,61.92 103.18,62.08
S$5274
  Bottom 0: 103.18,62.08 102.89,62.14
S$5275
  Bottom 0: 102.89,62.14 102.58,62.12
S$5276
  Bottom 0: 102.58,62.12 102.3,62.01
S$5277
  Bottom 0: 102.3,62.01 102.06,61.82
S$5278
  Bottom 0: 102.06,61.82 101.89,61.57
S$5279
  Bottom 0: 101.89,61.57 101.8,61.28
S$5280
  Bottom 0: 101.8,61.28 101.8,60.98
S$5281
  Bottom 0: 101.8,60.98 101.89,60.69
S$5282
  Bottom 0: 101.89,60.69 102.06,60.44
S$5283
  Bottom 0: 102.06,60.44 102.3,60.25
S$5284
  Bottom 0: 102.3,60.25 102.58,60.14
S$5285
  Bottom 0: 102.58,60.14 102.89,60.12
S$5286
  Bottom 0: 102.89,60.12 103.18,60.19
S$5287
  Bottom 0: 103.18,60.19 103.45,60.34
S$5288
  Bottom 0: 103.45,60.34 103.52,60.42
S$5289
  Bottom 0: 103.52,60.42 103.52,56.45
S$5290
  Bottom 0: 103.52,56.45 102.2,55.13
S$5291
  Bottom 0: 102.2,55.13 102.11,55.16
S$5292
  Bottom 0: 102.11,55.16 101.78,55.18
S$5293
  Bottom 0: 101.78,55.18 101.46,55.11
S$5294
  Bottom 0: 101.46,55.11 101.17,54.96
S$5295
  Bottom 0: 101.17,54.96 100.94,54.74
S$5296
  Bottom 0: 100.94,54.74 100.76,54.47
S$5297
  Bottom 0: 100.76,54.47 100.68,54.15
S$5298
  Bottom 0: 100.68,54.15 100.68,53.83
S$5299
  Bottom 0: 100.68,53.83 100.76,53.51
S$5300
  Bottom 0: 100.76,53.51 100.94,53.23
S$5301
  Bottom 0: 100.94,53.23 101.17,53.01
S$5302
  Bottom 0: 101.17,53.01 101.46,52.87
S$5303
  Bottom 0: 101.46,52.87 101.78,52.8
S$5304
  Bottom 0: 101.78,52.8 102.11,52.82
S$5305
  Bottom 0: 102.11,52.82 102.2,52.85
S$5306
  Bottom 0: 102.2,52.85 102.92,52.12
S$5307
  Bottom 0: 102.92,52.12 102.92,43.99
S$5308
  Bottom 0: 102.92,43.99 102.87,44.07
S$5309
  Bottom 0: 102.87,44.07 102.6,44.3
S$5310
  Bottom 0: 102.6,44.3 102.29,44.44
S$5311
  Bottom 0: 102.29,44.44 102.29,49.98
S$5312
  Bottom 0: 102.29,49.98 102.29,50.05
S$5313
  Bottom 0: 102.29,50.05 102.27,50.12
S$5314
  Bottom 0: 102.27,50.12 102.25,50.18
S$5315
  Bottom 0: 102.25,50.18 102.21,50.24
S$5316
  Bottom 0: 102.21,50.24 102.17,50.3
S$5317
  Bottom 0: 102.17,50.3 95.28,57.19
S$5318
  Bottom 0: 95.28,57.19 95.22,57.23
S$5319
  Bottom 0: 95.22,57.23 95.16,57.27
S$5320
  Bottom 0: 95.16,57.27 95.1,57.29
S$5321
  Bottom 0: 95.1,57.29 95.03,57.31
S$5322
  Bottom 0: 95.03,57.31 94.96,57.31
S$5323
  Bottom 0: 94.96,57.31 90.5,57.31
S$5324
  Bottom 0: 90.5,57.31 88.07,59.75
S$5325
  Bottom 0: 88.07,59.75 88.08,59.8
S$5326
  Bottom 0: 88.08,59.8 88.03,60.05
S$5327
  Bottom 0: 88.03,60.05 87.9,60.27
S$5328
  Bottom 0: 87.9,60.27 87.7,60.42
S$5329
  Bottom 0: 87.7,60.42 87.45,60.48
S$5330
  Bottom 0: 87.45,60.48 87.21,60.46
S$5331
  Bottom 0: 87.21,60.46 86.98,60.35
S$5332
  Bottom 0: 86.98,60.35 86.81,60.16
S$5333
  Bottom 0: 86.81,60.16 86.72,59.93
S$5334
  Bottom 0: 86.72,59.93 86.72,59.68
S$5335
  Bottom 0: 86.72,59.68 86.81,59.44
S$5336
  Bottom 0: 86.81,59.44 86.98,59.26
S$5337
  Bottom 0: 86.98,59.26 87.21,59.14
S$5338
  Bottom 0: 87.21,59.14 87.45,59.12
S$5339
  Bottom 0: 87.45,59.12 90,56.56
S$5340
  Bottom 0: 90,56.56 90.06,56.52
S$5341
  Bottom 0: 90.06,56.52 90.12,56.48
S$5342
  Bottom 0: 90.12,56.48 90.18,56.45
S$5343
  Bottom 0: 90.18,56.45 90.25,56.44
S$5344
  Bottom 0: 90.25,56.44 90.32,56.43
S$5345
  Bottom 0: 90.32,56.43 94.78,56.43
S$5346
  Bottom 0: 94.78,56.43 99.34,51.87
S$5347
  Bottom 0: 99.34,51.87 99.15,51.87
S$5348
  Bottom 0: 99.15,51.87 98.84,51.78
S$5349
  Bottom 0: 98.84,51.78 98.56,51.6
S$5350
  Bottom 0: 98.56,51.6 98.35,51.36
S$5351
  Bottom 0: 98.35,51.36 98.21,51.06
S$5352
  Bottom 0: 98.21,51.06 98.17,50.74
S$5353
  Bottom 0: 98.17,50.74 98.21,50.43
S$5354
  Bottom 0: 98.21,50.43 97.91,50.14
S$5355
  Bottom 0: 97.91,50.14 97.91,51.63
S$5356
  Bottom 0: 97.91,51.63 97.9,51.7
S$5357
  Bottom 0: 97.9,51.7 97.86,51.77
S$5358
  Bottom 0: 97.86,51.77 97.81,51.83
S$5359
  Bottom 0: 97.81,51.83 97.74,51.87
S$5360
  Bottom 0: 97.74,51.87 97.66,51.88
S$5361
  Bottom 0: 97.66,51.88 97.21,51.88
S$5362
  Bottom 0: 97.21,51.88 97.21,52.01
S$5363
  Bottom 0: 97.21,52.01 97.15,52.23
S$5364
  Bottom 0: 97.15,52.23 96.99,52.39
S$5365
  Bottom 0: 96.99,52.39 96.77,52.45
S$5366
  Bottom 0: 96.77,52.45 96.41,52.45
S$5367
  Bottom 0: 96.41,52.45 95.33,53.53
S$5368
  Bottom 0: 95.33,53.53 95.39,53.67
S$5369
  Bottom 0: 95.39,53.67 95.44,53.98
S$5370
  Bottom 0: 95.44,53.98 95.39,54.3
S$5371
  Bottom 0: 95.39,54.3 95.26,54.61
S$5372
  Bottom 0: 95.26,54.61 95.05,54.86
S$5373
  Bottom 0: 95.05,54.86 94.79,55.05
S$5374
  Bottom 0: 94.79,55.05 94.48,55.16
S$5375
  Bottom 0: 94.48,55.16 94.16,55.18
S$5376
  Bottom 0: 94.16,55.18 93.84,55.11
S$5377
  Bottom 0: 93.84,55.11 93.55,54.96
S$5378
  Bottom 0: 93.55,54.96 93.32,54.74
S$5379
  Bottom 0: 93.32,54.74 93.14,54.47
S$5380
  Bottom 0: 93.14,54.47 93.06,54.15
S$5381
  Bottom 0: 93.06,54.15 93.06,53.83
S$5382
  Bottom 0: 93.06,53.83 93.14,53.51
S$5383
  Bottom 0: 93.14,53.51 93.32,53.23
S$5384
  Bottom 0: 93.32,53.23 93.55,53.01
S$5385
  Bottom 0: 93.55,53.01 93.84,52.87
S$5386
  Bottom 0: 93.84,52.87 94.16,52.8
S$5387
  Bottom 0: 94.16,52.8 94.48,52.82
S$5388
  Bottom 0: 94.48,52.82 94.7,52.9
S$5389
  Bottom 0: 94.7,52.9 95.75,51.84
S$5390
  Bottom 0: 95.75,51.84 95.73,51.83
S$5391
  Bottom 0: 95.73,51.83 95.68,51.77
S$5392
  Bottom 0: 95.68,51.77 95.64,51.7
S$5393
  Bottom 0: 95.64,51.7 95.63,51.63
S$5394
  Bottom 0: 95.63,51.63 95.63,49.85
S$5395
  Bottom 0: 95.63,49.85 95.64,49.77
S$5396
  Bottom 0: 95.64,49.77 95.68,49.7
S$5397
  Bottom 0: 95.68,49.7 95.73,49.64
S$5398
  Bottom 0: 95.73,49.64 95.81,49.6
S$5399
  Bottom 0: 95.81,49.6 95.88,49.59
S$5400
  Bottom 0: 95.88,49.59 97.37,49.59
S$5401
  Bottom 0: 97.37,49.59 91.4,43.62
S$5402
  Bottom 0: 91.4,43.62 87.31,47.71
S$5403
  Bottom 0: 87.31,47.71 87.31,48.87
S$5404
  Bottom 0: 87.31,48.87 87.38,48.98
S$5405
  Bottom 0: 87.38,48.98 87.43,49.23
S$5406
  Bottom 0: 87.43,49.23 87.38,49.48
S$5407
  Bottom 0: 87.38,49.48 87.25,49.69
S$5408
  Bottom 0: 87.25,49.69 87.05,49.84
S$5409
  Bottom 0: 87.05,49.84 86.81,49.91
S$5410
  Bottom 0: 86.81,49.91 86.56,49.89
S$5411
  Bottom 0: 86.56,49.89 86.33,49.78
S$5412
  Bottom 0: 86.33,49.78 86.16,49.59
S$5413
  Bottom 0: 86.16,49.59 86.07,49.35
S$5414
  Bottom 0: 86.07,49.35 86.07,49.1
S$5415
  Bottom 0: 86.07,49.1 86.16,48.87
S$5416
  Bottom 0: 86.16,48.87 86.17,48.85
S$5417
  Bottom 0: 86.17,48.85 86.17,47.48
S$5418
